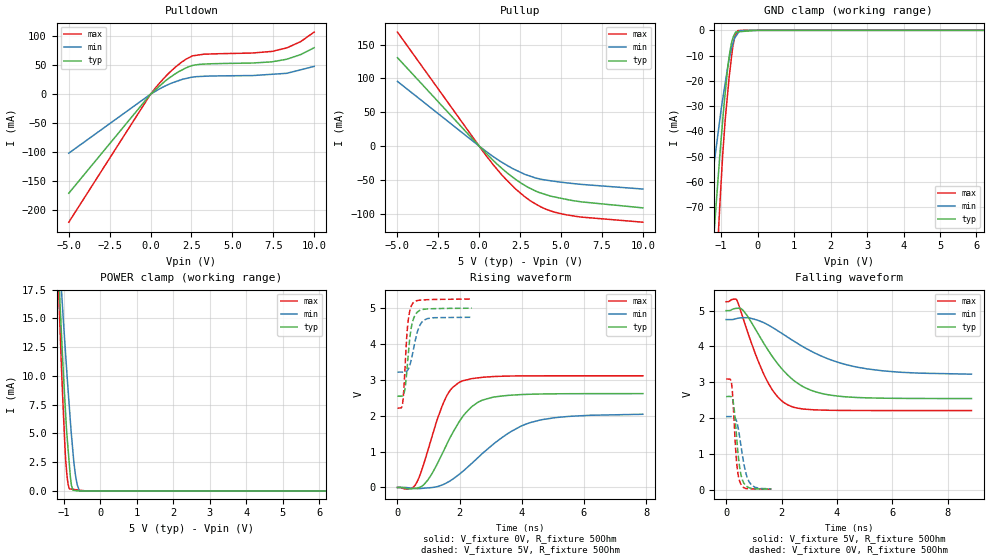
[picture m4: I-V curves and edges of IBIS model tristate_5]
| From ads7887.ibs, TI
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|   tristate_5 Model
[Model]   tristate_5
Model_type   3-state
Polarity   Non-Inverting
Vmeas = 2.5
Vref  = 2.5
Cref  = 50pF
Rref  = 50
|   typ   min   max
|   (nom PVT)   (Fast PVT)   (slow PVT)
|C_comp from frequency method(F=25MHz)
|Average
|C_comp   3.815e-12   3.125e-12   4.770e-12
|ON state : BUFFER OUTPUT TURNED HIGH
|C_comp   3.815e-12   3.125e-12   4.770e-12
|OFF state: BUFFER IN HIGH IMPEDANCE
|C_comp   2.439e-12   1.809e-12   2.939e-12
|C_comp from L-C Tank method(L=1nH)
C_comp   1.914e-12   1.472e-12   2.371e-12
|ON state : BUFFER OUTPUT TURNED HIGH
|Resonant Frequency(Hz)   3.640e09   4.150e09   3.270e09
|C_comp   1.914e-12   1.472e-12   2.371e-12
|OFF state: BUFFER IN HIGH IMPEDANCE
|Resonant Frequency(Hz)   3.670e09   4.210e09   3.290e09
|C_comp   1.883e-12   1.431e-12   2.343e-12
| Where nom  PVT is Nominal Process,  5V,  28C
|   Fast PVT is Strong Process,   5.25V,  -40C
|   Slow PVT is Weak Process,   4.75V,  128C
[Voltage Range]   5   4.75   5.25
|Ambient Temperature   25   125   -40
|Junction Temperature
[Temperature Range]   28   128   -40
[Pullup Reference]   5   4.75   5.25
[Pulldown Reference]   0   0   0
[Power Clamp Reference]   5   4.75   5.25
[GND Clamp Reference]   0   0   0
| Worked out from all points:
|   slope of the pulldown table from 0 to 0.75 V, typ, clamps not added: 39.5 ohm
|   slope of the pullup table from 0 to 0.75 V, typ, clamps not added: 40.5 ohm
|   GND clamp passes 1 mA (typ) near -0.61 V on its own axis
|   POWER clamp passes 1 mA (typ) near -0.81 V on its own axis
|   falling waveform, V_fixture 5V, R_fixture 50Ohm: 20-80 % time 1.43ns typ, 2.3ns min, 967ps max; typ from 5 V to 2.54 V
|   rising waveform, V_fixture 0V, R_fixture 50Ohm: 20-80 % time 1.01ns typ, 1.76ns min, 715ps max; typ from 0 V to 2.61 V
|   rising waveform, V_fixture 5V, R_fixture 50Ohm: 20-80 % time 176ps typ, 247ps min, 134ps max; typ from 2.54 V to 4.99 V
|   falling waveform, V_fixture 0V, R_fixture 50Ohm: 20-80 % time 194ps typ, 272ps min, 148ps max; typ from 2.6 V to 0.015 V
[Pulldown]
|   Voltage   I(typ)   I(min)   I(max)
-5V       -170.3mA   -101.4mA   -220.1mA
0V        0A         0A         0A
885.2mV   22.39mA    13.93mA    29.49mA
1.526V    35.31mA    21.4mA     46.68mA
1.904V    41.35mA    25.11mA    55.09mA
2.55V     49.18mA    29.28mA    65.77mA
3.232V    51.63mA    30.69mA    68.64mA
6.266V    53.6mA     32.02mA    70.83mA
7.427V    55.6mA     34.18mA    73.52mA
8.34V     60.16mA    35.97mA    79.66mA
9.175V    67.99mA    41.89mA    90.36mA
10V       79.81mA    47.75mA    106.7mA
[GND Clamp]
|   Voltage   I(typ)   I(min)   I(max)
-5V       -955.7mA   -644.6mA   -1.294A
-1.445V   -131.7mA   -83.71mA   -189.2mA
-1.246V   -90.23mA   -58.71mA   -129mA
-1.042V   -50.48mA   -35.91mA   -70.56mA
-957.5mV  -35.71mA   -27.27mA   -49.3mA
-894.5mV  -25.64mA   -21.43mA   -36.51mA
-779mV    -10.1mA    -11.45mA   -18.3mA
-684.5mV  -3.325mA   -5.578mA   -6.835mA
-621.5mV  -1.218mA   -2.892mA   -2.28mA
-542.7mV  -585.3uA   -1.21mA    -118.4uA
-183.5mV  -194.3uA   0A         0A
10V       0A         0A         0A
[Pullup]
|   Voltage   I(typ)   I(min)   I(max)
-5V       130.7mA    95.63mA    168.4mA
507.2mV   -12.52mA   -9.326mA   -16.64mA
1.526V    -35.81mA   -25.78mA   -46.26mA
2.166V    -48.01mA   -34.47mA   -61.91mA
2.78V     -57.84mA   -41.5mA    -74.57mA
3.232V    -63.67mA   -45.23mA   -82.33mA
3.778V    -69.25mA   -48.83mA   -89.85mA
4.424V    -73.99mA   -51.29mA   -96.03mA
5.154V    -77.67mA   -53.57mA   -100.5mA
6.256V    -82.24mA   -56.44mA   -104.7mA
10V       -91.04mA   -63.27mA   -112.2mA
[POWER Clamp]
|   Voltage   I(typ)   I(min)   I(max)
-5V       174.8mA    150.8mA    199.2mA
-1.246V   25.98mA    26.72mA    26.49mA
-1.068V   13.87mA    17.63mA    10.97mA
-1.036V   11.73mA    16.02mA    8.559mA
-962.7mV  7.419mA    12.46mA    3.445mA
-910.3mV  4.699mA    9.99mA     1.236mA
-878.8mV  3.469mA    8.607mA    509uA
-820mV    1.224mA    6.028mA    167.5uA
-750mV    64.66uA    3.396mA    139.8uA
-682.3mV  33.26uA    1.398mA    113.1uA
-573mV    0A         5.448uA    69.96uA
10V       0A         0A         0A
[Ramp]
R_load = 50
|   typ   min   max
dV/dt_r   1.56813/1.00981e-09   1.22822/1.76859e-09   1.86481/7.11916e-10
dV/dt_f   1.47561/1.43075e-09   0.922542/2.33815e-09   1.82565/9.67874e-10
[Falling Waveform]
V_fixture = 5V
V_fixture_min = 4.75V
V_fixture_max = 5.25V
R_fixture = 50Ohm
|   Time   V(typ)   V(min)   V(max)
0s        5V         4.75V      5.25V
383ps     5.064V     4.781V     5.302V
641ps     4.982V     4.803V     4.718V
1.103ns   4.421V     4.741V     3.695V
1.419ns   4.012V     4.64V      3.127V
1.871ns   3.506V     4.433V     2.582V
2.254ns   3.176V     4.241V     2.355V
3.159ns   2.747V     3.83V      2.229V
4.734ns   2.572V     3.42V      2.209V
8.852ns   2.542V     3.224V     2.207V
[Rising Waveform]
V_fixture = 0V
V_fixture_min = 0V
V_fixture_max = 0V
R_fixture = 50Ohm
|   Time   V(typ)   V(min)   V(max)
0s        1.456nV    2.446nV    1.291nV
578ps     -20.7mV    -31.4mV    73.64mV
983ps     213.1mV    -11.49mV   1.042V
1.479ns   1.005V     83.3mV     2.353V
1.715ns   1.422V     194.8mV    2.724V
2.015ns   1.869V     384.5mV    2.938V
2.716ns   2.425V     932.8mV    3.065V
3.515ns   2.56V      1.48V      3.1V
4.268ns   2.595V     1.804V     3.108V
7.896ns   2.613V     2.038V     3.109V
[Rising Waveform]
V_fixture = 5V
V_fixture_min = 4.75V
V_fixture_max = 5.25V
R_fixture = 50Ohm
|   Time   V(typ)   V(min)   V(max)
0s        2.541V     3.212V     2.207V
168ps     2.55V      3.212V     2.355V
244ps     2.763V     3.213V     3.34V
293ps     3.142V     3.231V     4.121V
334ps     3.555V     3.272V     4.557V
406ps     4.218V     3.427V     4.943V
486ps     4.609V     3.721V     5.119V
657ps     4.894V     4.378V     5.207V
861ps     4.963V     4.662V     5.223V
2.395ns   4.991V     4.739V     5.245V
[Falling Waveform]
V_fixture = 0V
V_fixture_min = 0V
V_fixture_max = 0V
R_fixture = 50Ohm
|   Time   V(typ)   V(min)   V(max)
0s        2.6V       2.04V      3.089V
146ps     2.601V     2.04V      3.087V
206ps     2.576V     2.04V      2.904V
278ps     2.337V     2.03V      2.059V
378ps     1.475V     1.91V      769.5mV
441ps     924.2mV    1.694V     379.5mV
507ps     526.2mV    1.372V     192.8mV
698ps     117.1mV    505.9mV    31.53mV
836ps     49.01mV    206.5mV    17.51mV
1.632ns   14.54mV    19mV       10.04mV
